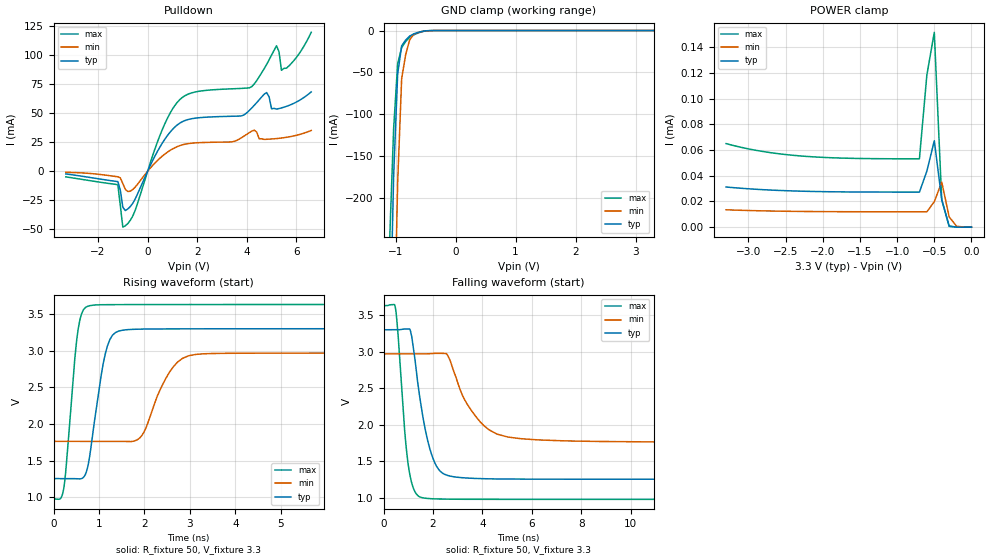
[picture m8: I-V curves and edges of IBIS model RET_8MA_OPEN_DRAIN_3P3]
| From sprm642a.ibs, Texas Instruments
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|   Model Cell RET_8MA_OPEN_DRAIN_3P3
|RET_8MA_OPEN_DRAIN_3P3
[Model]   RET_8MA_OPEN_DRAIN_3P3
Model_type   I/O_open_drain
Polarity   Inverting
Enable   Active-Low
Vinl =  0.8
Vinh =  2
Cref =  15.0000pF
Rref =  100.0000M
Vref =  0V
Vmeas =  1.65
C_comp   5.345208p   4.561426p   6.022817p
[Model Spec]
Vinl   0.8   0.8   0.8
Vinh   2   2   2
[Temperature Range]   25   155   -40
[Voltage Range]   3.3   2.97   3.63
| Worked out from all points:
|   slope of the pulldown table from 0 to 0.495 V, typ, clamps not added: 23.8 ohm
|   GND clamp passes 1 mA (typ) near -0.55 V on its own axis
|   rising waveform, R_fixture 50, V_fixture 3.3: 20-80 % time 297ps typ, 507ps min, 211ps max; typ from 1.26 V to 3.3 V
|   falling waveform, R_fixture 50, V_fixture 3.3: 20-80 % time 607ps typ, 1.17ns min, 363ps max; typ from 3.3 V to 1.26 V
| Nom Voltages:
|   BIASFET=3.3, VDD=1.2, VDDS=3.3, VSS=0
| Min Voltages:
|   BIASFET=2.97, VDD=1.08, VDDS=2.97, VSS=0
| Max Voltages:
|   BIASFET=3.63, VDD=1.32, VDDS=3.63, VSS=0
[POWER_clamp]
|   voltage   I(typ)   I(min)   I(max)
-3.3V     31.22uA    13.5uA     64.95uA
-2.8V     29.13uA    12.67uA    58.77uA
-2.3V     27.98uA    12.22uA    55.36uA
-1.7V     27.4uA     12.01uA    53.62uA
-700mV    27.24uA    11.95uA    53.12uA
-600mV    43.52uA    11.94uA    118.2uA
-500mV    67.2uA     19.79uA    151.5uA
-400mV    21.58uA    35.09uA    21.1uA
-300mV    927.4nA    7.958uA    611.4nA
-200mV    28.93nA    716.3nA    11.51nA
0V        696.9pA    39.48nA    568.3pA
[Pulldown]
|   voltage   I(typ)   I(min)   I(max)
-3.3V     -2.325mA   -885.1uA   -4.829mA
-1.2V     -8.9mA     -4.742mA   -11.78mA
-1V       -30.94mA   -10.56mA   -48.07mA
-900mV    -33.77mA   -15.53mA   -46.9mA
-500mV    -23.82mA   -13.61mA   -33.55mA
600mV     24.46mA    13.16mA    36.18mA
1.3V      41.39mA    22.04mA    61.62mA
4.2V      54.39mA    34.49mA    72.77mA
4.8V      67.66mA    27.49mA    91.8mA
5.2V      53.41mA    28.11mA    107.8mA
5.4V      54.46mA    28.58mA    86.79mA
6.6V      68.25mA    35.07mA    119.5mA
[GND_clamp]
|   voltage   I(typ)   I(min)   I(max)
-3.3V     -16.36A    -15.08A    -17.18A
-1.1V     -382.1mA   -717.8mA   -250.1mA
-1.033V   -173.3mA   -402.2mA   -116.4mA
-966.7mV  -52.02mA   -182.1mA   -39.81mA
-900mV    -18.21mA   -57.43mA   -20.34mA
-833.3mV  -11.36mA   -28.88mA   -13.17mA
-766.7mV  -6.618mA   -11.27mA   -8.134mA
-700mV    -3.983mA   -4.59mA    -5.247mA
-500mV    -328.3uA   -481.4uA   -374.5uA
-366.7mV  -15.94uA   -50.74uA   -14.83uA
3.3V      696.9pA    15.84uA    426.1pA
[Ramp]
| variable   typ   min   max
dV/dt_f  1.2327083/0.6089555n 0.72801541/1.1737387n   1.597487/0.3638698n
dV/dt_r  1.2367288/0.5366087n  0.8469789/1.2334714n  1.5908665/0.32475913n
R_load = 50
[Rising Waveform]
R_fixture = 50
V_fixture = 3.3
V_fixture_min = 2.97
V_fixture_max = 3.63
|   time   V(typ)   V(min)   V(max)
0s        1.258V     1.765V     982mV
224.7ps   1.258V     1.765V     1.121V
543.4ps   1.253V     1.765V     3.298V
790.9ps   1.546V     1.765V     3.613V
1.139ns   2.958V     1.765V     3.628V
1.502ns   3.278V     1.765V     3.629V
1.938ns   3.295V     1.841V     3.629V
2.552ns   3.298V     2.709V     3.63V
3.132ns   3.299V     2.95V      3.63V
20.01ns   3.3V       2.97V      3.63V
[Falling Waveform]
R_fixture = 50
V_fixture = 3.3
V_fixture_min = 2.97
V_fixture_max = 3.63
|   time   V(typ)   V(min)   V(max)
0s        3.3V       2.97V      3.63V
468.7ps   3.3V       2.97V      3.613V
956.5ps   3.311V     2.97V      1.555V
1.14ns    3.202V     2.97V      1.201V
1.441ns   2.428V     2.97V      1.019V
1.983ns   1.554V     2.977V     990.1mV
2.772ns   1.294V     2.796V     984.4mV
3.81ns    1.267V     2.081V     982.9mV
5.03ns    1.26V      1.834V     982.7mV
20.01ns   1.258V     1.765V     982.8mV
